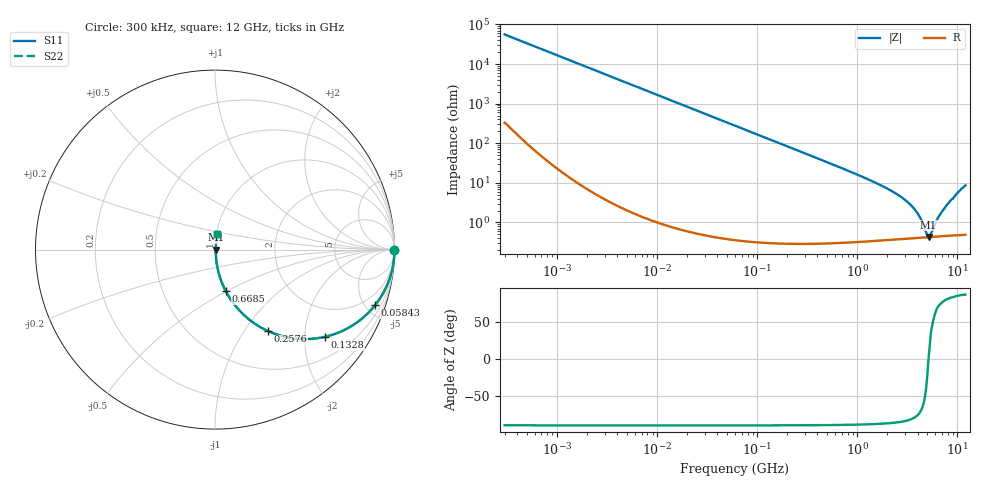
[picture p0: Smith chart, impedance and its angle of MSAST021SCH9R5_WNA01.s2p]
! MSAST021SCH9R5_WNA01  S-PARAMETER MODEL  ( General Type )
! Model Generated by TAIYO YUDEN Corporation (http://www.ty-top.com)
! Version 2.0
! TAIYO YUDEN Control No. 181101
! Copyright(c) 2015 TAIYO YUDEN CO.,LTD. All Rights Reserved.
! Product Description (link to TY-COMPAS)
! https://ds.yuden.co.jp/TYCOMPAS/or/detail?pn=MSAST021SCH9R5CWNA01&u=M
! Products Name : Multilayer Ceramic Capacitors
! Characteristics :
!  Capacitance : 9.5 pF , Rated Voltage : 25V , TCC : CH / C0H
!  Case Size : 0.25 x 0.125 / 0.0098 x 0.0049 [mm/inch] , Thickness : 0.125 / 0.0049 [mm/inch]
!  (Conditions: Temperature = 25 degC , DC Bias Current/Voltage = 0A / 0V)
! External Node Assignments :
!  1  o---| |---o  2
! GND o---------o GND
! Frequency Range : 0.3MHz  -  12000MHz  [ 401 STEP ]
# MHz S RI R 50
! Freq[MHz].  S11 Real  S11 Imag  S21 Real  S21 Imag  S12 Real  S12 Imag  S22 Real  S22 Imag
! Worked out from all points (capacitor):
!   401 points, 300 kHz to 12 GHz, reference 50 ohm
!   read as one part in series: C = 9.5 pF near 316.3 kHz
!   lowest |Z| = 427 mohm at 5.141 GHz (marker M1)
!   series resonance near 5.136 GHz, so ESL is about 100 pH
!   S11 on the Smith chart (normalised r, x): 300 kHz: open; 58.43 MHz: 1.01, -5.73; 132.8 MHz: 1.01, -2.52; 257.6 MHz: 1.01, -1.30; 668.5 MHz: 1.01, -0.49; 12 GHz: 1.01, +0.17
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0.3  1 -0.00179  1.38e-05 0.00179  1.38e-05 0.00179  1 -0.00179
1.769972  0.9999 -0.0106  0.000121 0.0106  0.000121 0.0106  0.9999 -0.0106
10.44266  0.9961 -0.0621  0.00391 0.0621  0.00391 0.0621  0.9961 -0.0621
25.70316  0.9769 -0.1499  0.0231 0.1499  0.0231 0.1499  0.9769 -0.1499
58.43137  0.8912 -0.3107  0.1088 0.3107  0.1088 0.3107  0.8912 -0.3107
60  0.886 -0.3172  0.114 0.3172  0.114 0.3172  0.886 -0.3172
89.27472  0.7783 -0.4145  0.2217 0.4145  0.2217 0.4145  0.7783 -0.4145
132.8329  0.6134 -0.4858  0.3866 0.4858  0.3866 0.4858  0.6134 -0.4858
257.5933  0.297 -0.4547  0.703 0.4547  0.703 0.4547  0.297 -0.4547
353.9943  0.1831 -0.3837  0.8169 0.3837  0.8169 0.3837  0.1831 -0.3837
668.5285  0.0597 -0.2309  0.9403 0.2309  0.9403 0.2309  0.0597 -0.2309
2088.533  0.00802 -0.0662  0.992 0.0662  0.992 0.0662  0.00802 -0.0662
2870.14  0.00541 -0.0398  0.9946 0.0398  0.9946 0.0398  0.00541 -0.0398
3642.919  0.00451 -0.0227  0.9955 0.0227  0.9955 0.0227  0.00451 -0.0227
4158.869  0.00428 -0.0137  0.9957 0.0137  0.9957 0.0137  0.00428 -0.0137
4875.354  0.00422 -0.00336  0.9958 0.00336  0.9958 0.00336  0.00422 -0.00336
5140.631  0.00425 5.59e-05  0.9958 -5.59e-05  0.9958 -5.59e-05  0.00425 5.59e-05
5420.343  0.0043 0.00301  0.9957 -0.00301  0.9957 -0.00301  0.0043 0.00301
6354.153  0.00455 0.012  0.9954 -0.012  0.9954 -0.012  0.00455 0.012
7448.838  0.00503 0.0225  0.995 -0.0225  0.995 -0.0225  0.00503 0.0225
10236.47  0.00817 0.0582  0.9918 -0.0582  0.9918 -0.0582  0.00817 0.0582
12000  0.0121 0.0845  0.9879 -0.0845  0.9879 -0.0845  0.0121 0.0845
